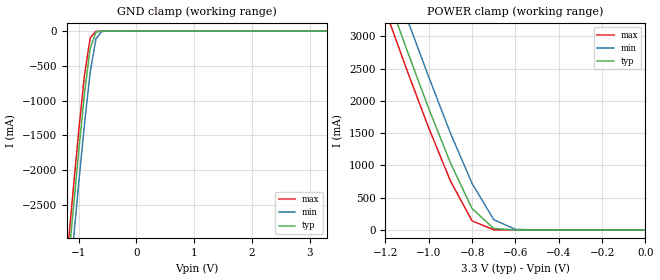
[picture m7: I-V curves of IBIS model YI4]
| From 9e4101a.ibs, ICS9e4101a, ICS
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|   Model YI4
[Model]   YI4
Model_type   Input
Polarity   Inverting
Vinl =   0.80V
Vinh =   2.00V
C_comp   5.50pF   5.00pF   6.00pF
[Temperature Range]   27.00   70.00   0.000
[Voltage Range]   3.30V   3.00V   3.70V
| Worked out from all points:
|   GND clamp passes 1 mA (typ) near -0.60 V on its own axis
|   POWER clamp passes 1 mA (typ) near -0.60 V on its own axis
[GND_clamp]
| voltage   I(typ)   I(min)   I(max)
-3.3V     -24.05A    -24.48A    -23.79A
-1.2V     -3.55A     -4.02A     -3.26A
-1.1V     -2.63A     -3.1A      -2.34A
-1V       -1.74A     -2.2A      -1.45A
-900mV    -910mA     -1.35A     -640mA
-800mV    -250mA     -590mA     -96.84mA
-700mV    -14.58mA   -110mA     -3.87mA
-600mV    -880uA     -5.82mA    -450uA
-500mV    -88.51uA   -350uA     -45.1uA
3.3V      130pA      470nA      90.8pA
[POWER_clamp]
| voltage   I(typ)   I(min)   I(max)
-3.3V     24.22A     24.67A     23.94A
-1.2V     3.71A      4.2A       3.4A
-1.1V     2.78A      3.27A      2.47A
-1V       1.88A      2.37A      1.58A
-900mV    1.04A      1.5A       760mA
-800mV    330mA      720mA      140mA
-700mV    23.26mA    160mA      3.86mA
-600mV    560uA      9.41mA     65.3uA
0V        130pA      310pA      130pA
